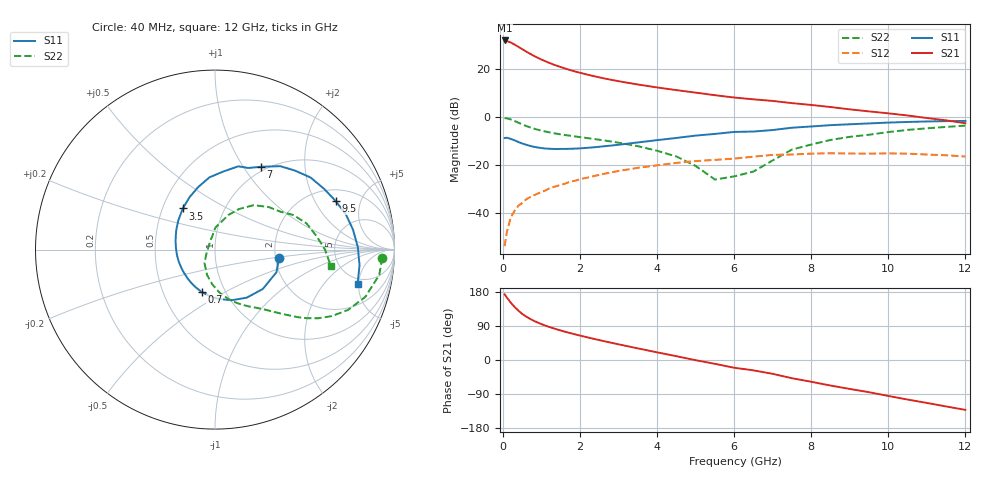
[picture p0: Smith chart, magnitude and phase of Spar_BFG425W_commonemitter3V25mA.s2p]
! Filename: 325bfg425.001
! BFG425W Field C1
! V1=8.521E-001V,V2=3.000E+000V, I1=3.334E-004A, I2=2.502E-002A
# GHz  S  MA  R 50
!  S11  S21  S12  S22
!Freq(GHz)  Mag  Ang  Mag  Ang  Mag  Ang  Mag  Ang
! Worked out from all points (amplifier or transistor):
!   44 points, 40 MHz to 12 GHz, reference 50 ohm
!   highest |S21| = 31.8 dB at 40 MHz (marker M1)
!   |S21| within 3 dB of that: start of sweep to 433.1 MHz
!   unconditionally stable (mu >= 1): 1.238 GHz to end of sweep
!   at 700 MHz: K = 0.80, MSG = 29.9 dB, |S12| = -33.6 dB
!   at 2.4 GHz: K = 1.16, MAG = 18.3 dB, |S12| = -24.6 dB
!   at 12 GHz: K = 1.34, MAG = 3.4 dB, |S12| = -16.6 dB
!   S11 on the Smith chart (normalised r, x): 40 MHz: 2.09, -0.23; 700 MHz: 0.78, -0.39; 3.5 GHz: 0.63, +0.32; 7 GHz: 0.94, +1.21; 9.5 GHz: 2.64, +3.00; 12 GHz: 4.27, -4.86
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0.04  0.36 -7.5  38.91 173.1  0.002 74.5  0.933 -2.8
0.1  0.365 -20.3  37.79 164.8  0.004 82.4  0.926 -8.8
0.2  0.345 -39.5  35.24 151.2  0.008 76.2  0.878 -17.5
0.3  0.321 -56.5  31.93 139.8  0.011 72.1  0.814 -24.4
0.4  0.297 -71.8  28.6 130.0  0.014 69.4  0.749 -29.6
0.5  0.276 -85.6  25.54 121.4  0.016 66.6  0.691 -33.6
0.6  0.26 -97.2  22.83 114.5  0.019 65.0  0.641 -36.6
0.7  0.247 -107.6  20.54 108.7  0.021 63.8  0.6 -39.0
0.9  0.228 -125.3  16.95 98.8  0.025 62.4  0.536 -42.6
1.2  0.215 -146.0  13.26 87.2  0.032 60.4  0.473 -47.0
1.6  0.213 -167.8  10.19 74.9  0.04 57.5  0.416 -52.3
2.2  0.225 167.4  7.498 59.5  0.054 51.6  0.357 -61.1
2.8  0.25 147.4  5.897 45.7  0.069 44.6  0.305 -70.9
3.5  0.291 128.1  4.693 30.6  0.086 35.1  0.243 -83.7
4.5  0.361 105.0  3.587 10.0  0.109 20.1  0.148 -107.4
5.5  0.438 83.8  2.808 -10.1  0.126 4.4  0.049 -160.6
6.5  0.491 67.9  2.306 -27.4  0.147 -8.0  0.072 103.8
7  0.528 60.9  2.132 -36.6  0.16 -15.7  0.123 89.0
8.5  0.667 37.0  1.593 -67.4  0.173 -45.0  0.328 49.0
9.5  0.725 21.8  1.291 -85.0  0.17 -61.7  0.421 30.1
10.5  0.777 8.2  1.061 -104.4  0.17 -80.3  0.531 15.9
12  0.817 -13.4  0.732 -131.6  0.148 -110.1  0.652 -8.1
